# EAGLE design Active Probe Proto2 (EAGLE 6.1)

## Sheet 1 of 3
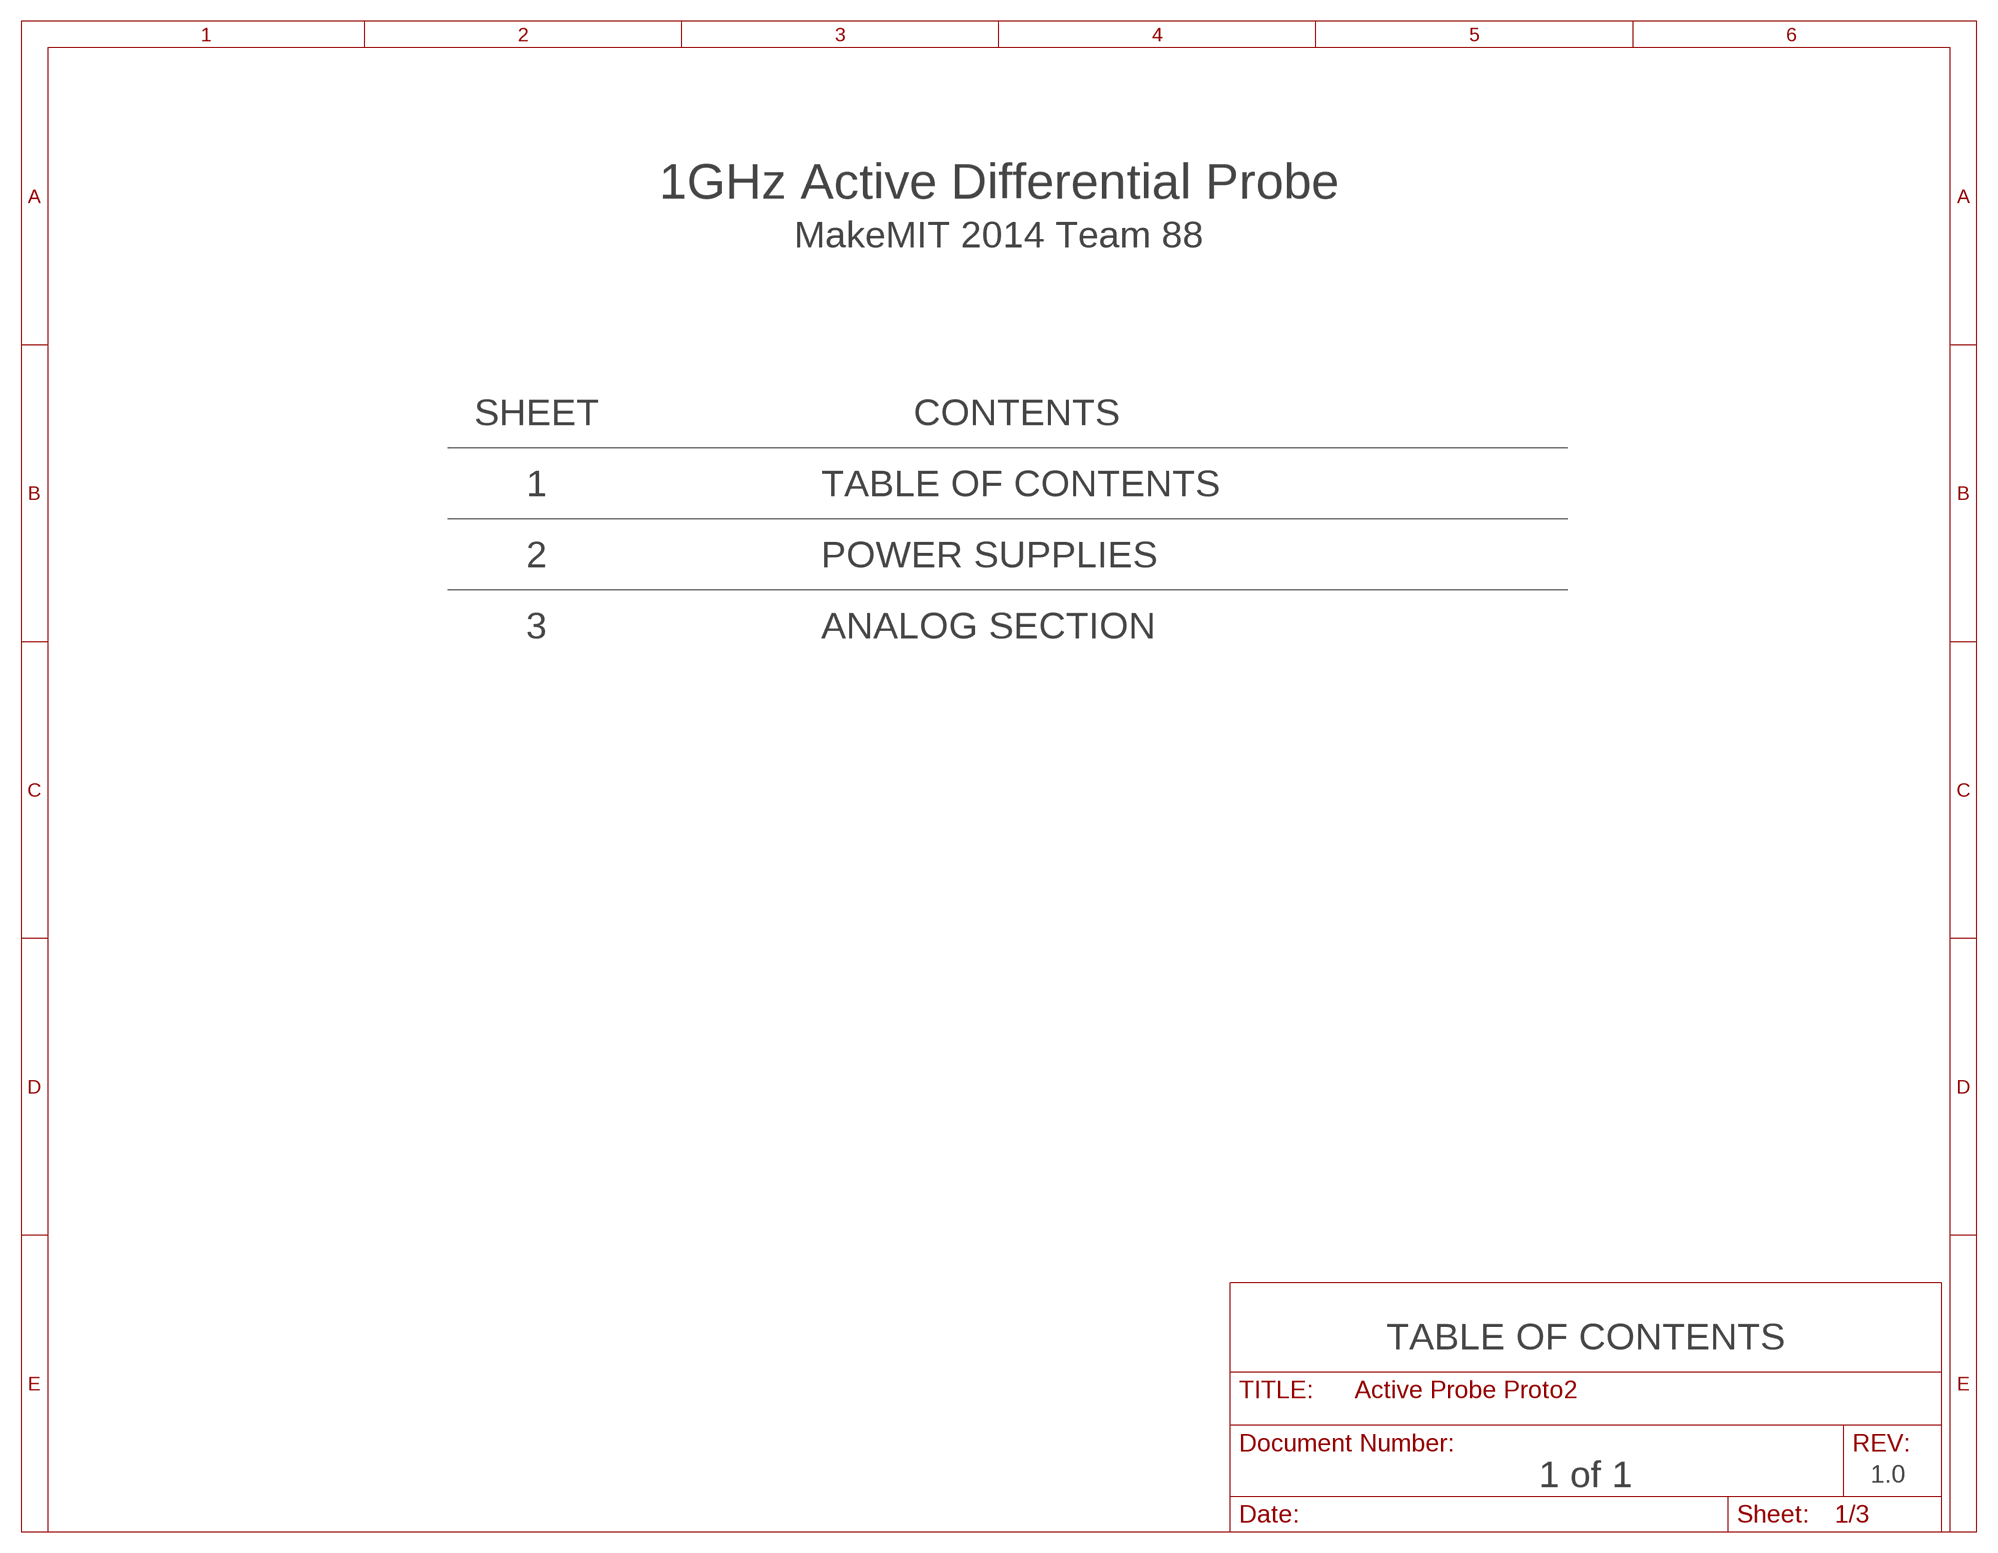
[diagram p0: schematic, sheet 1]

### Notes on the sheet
- 1GHz Active Differential Probe
- MakeMIT 2014 Team 88
- SHEET | CONTENTS
- 1 | TABLE OF CONTENTS
- 2 | POWER SUPPLIES
- 3 | ANALOG SECTION
- TABLE OF CONTENTS
- 1 of 1 | 1.0

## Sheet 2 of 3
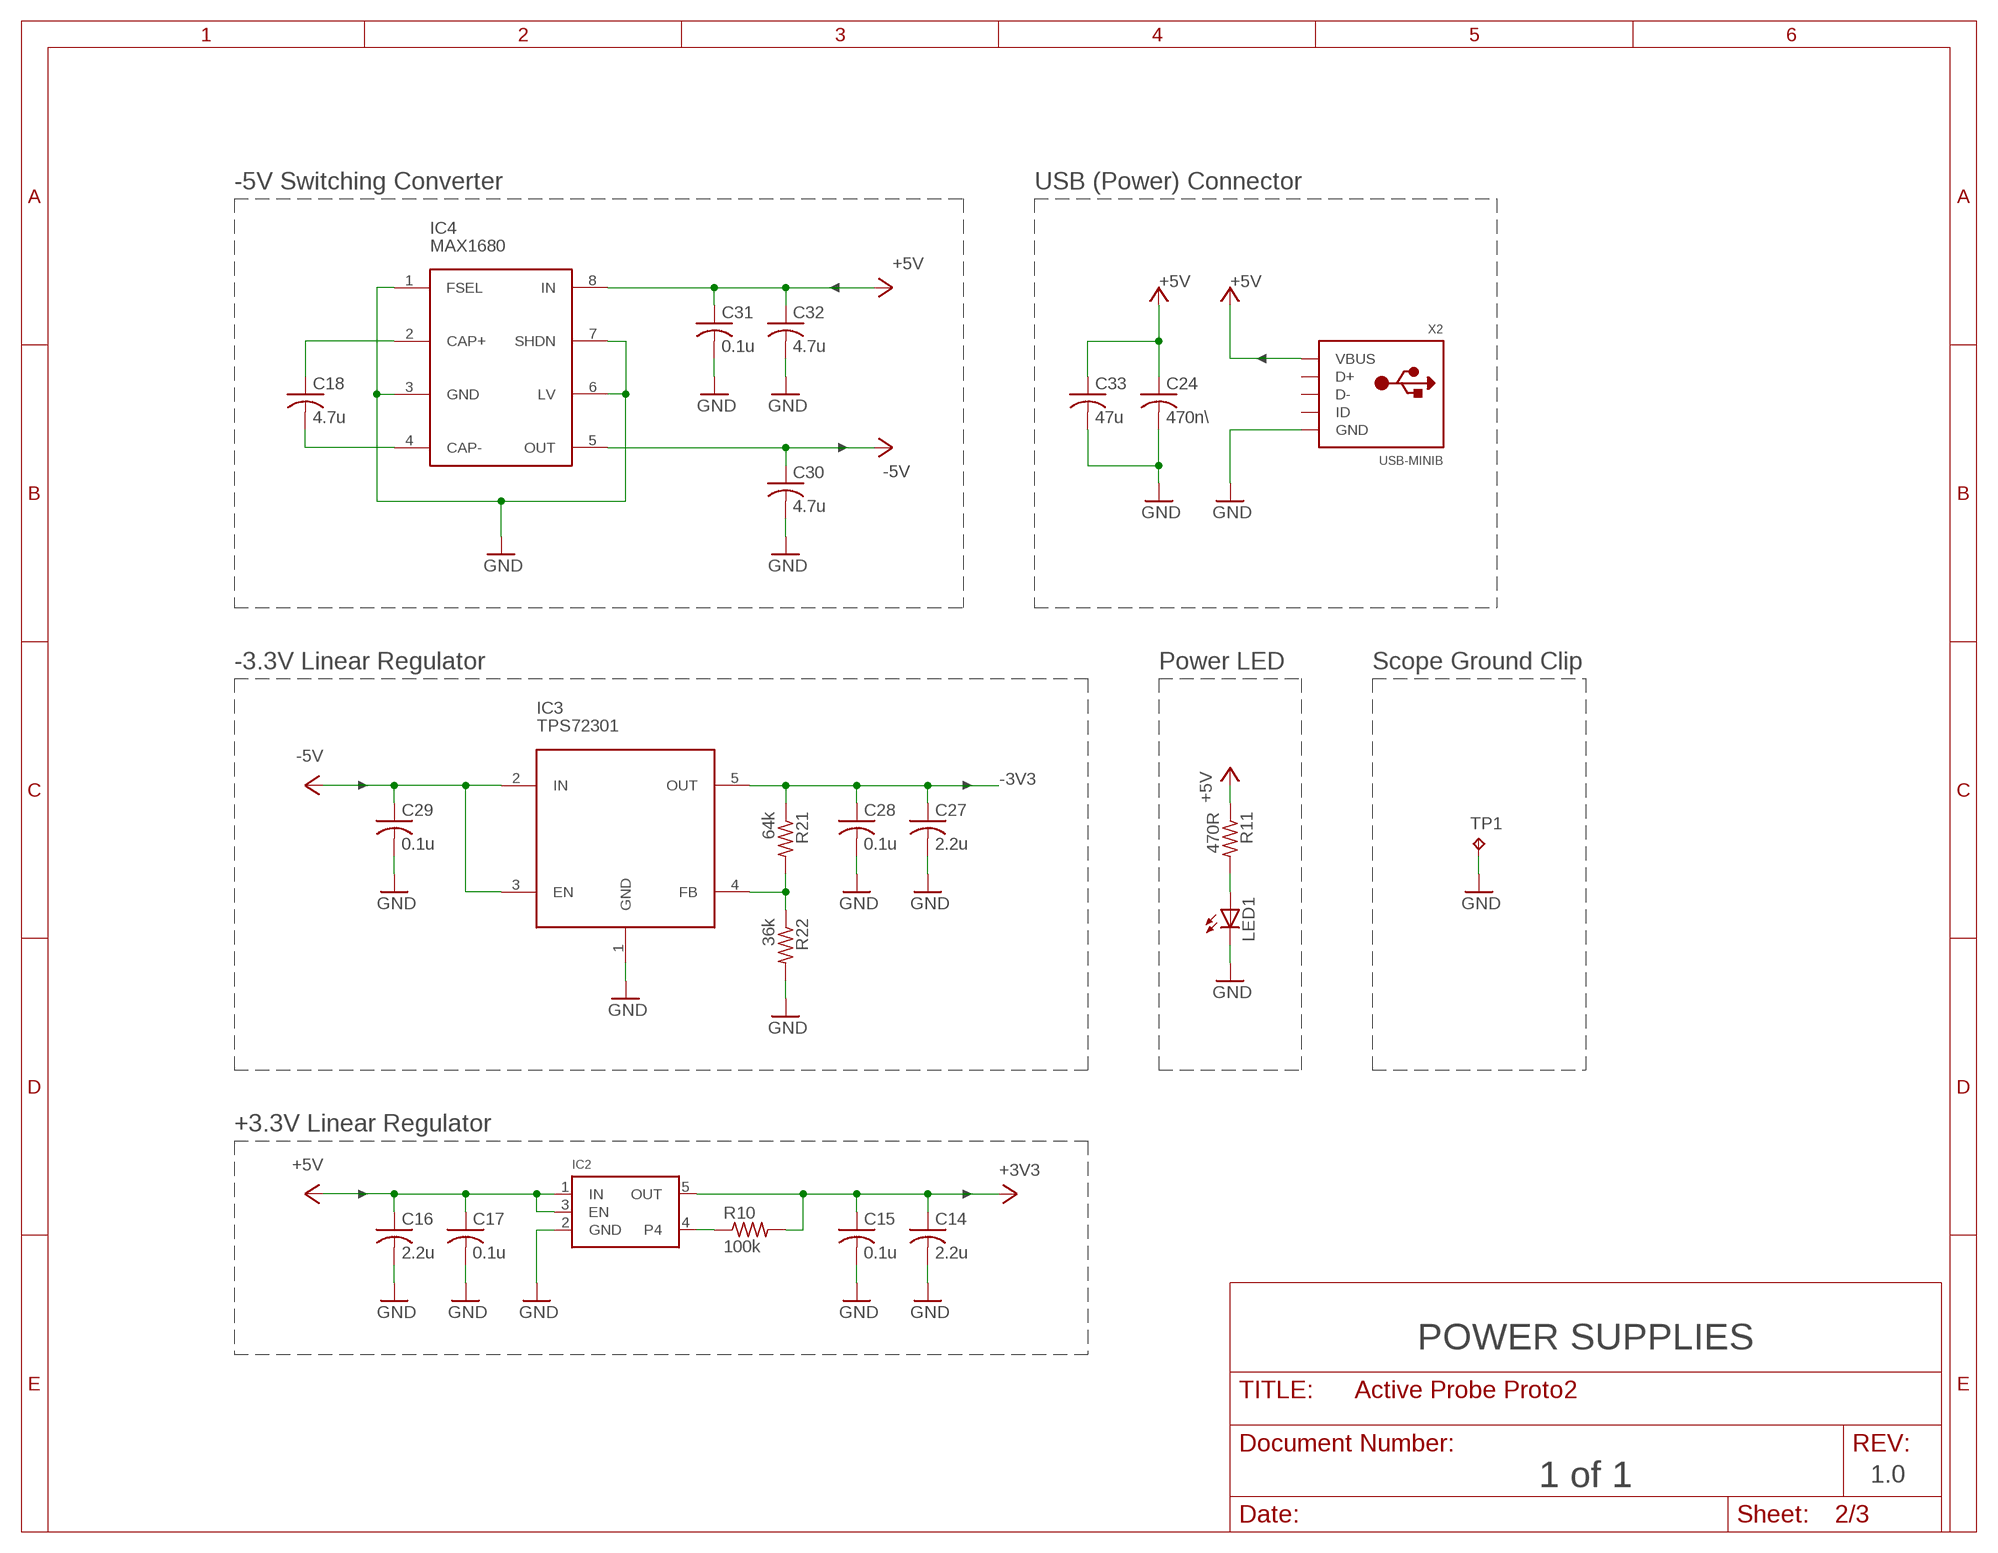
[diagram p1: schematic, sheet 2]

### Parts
C14  2.2u  C-USC0603  [C0603]
C15  0.1u  C-USC0603  [C0603]
C16  2.2u  C-USC0603  [C0603]
C17  0.1u  C-USC0603  [C0603]
C18  4.7u  C-USC0603  [C0603]
C24  470n\  C-USC0603  [C0603]
C27  2.2u  C-USC0603  [C0603]
C28  0.1u  C-USC0603  [C0603]
C29  0.1u  C-USC0603  [C0603]
C30  4.7u  C-USC0603  [C0603]
C31  0.1u  C-USC0603  [C0603]
C32  4.7u  C-USC0603  [C0603]
C33  47u  C-USC1206  [C1206]
IC2  VREG_SOT23-5  [SOT23-5]
IC3  TPS72301  [SOT23-5L]
IC4  MAX1680  MAX1680/1  [SO8]
LED1  LED3MM  [LED3MM]
R10  100k  R-US_R0603  [R0603]
R11  470R  R-US_R0805  [R0805]
R21  64k  R-US_R0603  [R0603]
R22  36k  R-US_R0603  [R0603]
TP1  TPTP20SQ  [TP20SQ]
X2  USB-MINIB  USBMINIB  [USB-MINIB]

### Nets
+3V3: C14.1 C15.1 IC2.5(OUT) R10.2 ; also sheet 3
+5V: C16.1 C17.1 C24.1 C31.1 C32.1 C33.1 IC2.1(IN) IC2.3(EN) IC4.8(IN) R11.1 X2.VBUS ; also sheet 3
-3V3: C27.1 C28.1 IC3.5(OUT) R21.1 ; also sheet 3
-5V: C29.1 C30.1 IC3.2(IN) IC3.3(EN) IC4.5(OUT)
GND: C14.2 C15.2 C16.2 C17.2 C24.2 C27.2 C28.2 C29.2 C30.2 C31.2 C32.2 C33.2 IC2.2(GND) IC3.1(GND) IC4.1(FSEL) IC4.3(GND) IC4.6(LV) IC4.7(SHDN) LED1.K(C) R22.2 TP1.TP X2.GND ; also sheet 3
N$4: IC2.4 R10.1
N$11: LED1.A R11.2
N$14: C18.2 IC4.4(CAP-)
N$15: C18.1 IC4.2(CAP+)
N$19: IC3.4(FB) R21.2 R22.1
Unconnected: X2.D+ X2.D- X2.ID

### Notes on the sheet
- -5V Switching Converter | USB (Power) Connector
- -3.3V Linear Regulator | Power LED | Scope Ground Clip
- +3.3V Linear Regulator
- POWER SUPPLIES
- 1 of 1 | 1.0

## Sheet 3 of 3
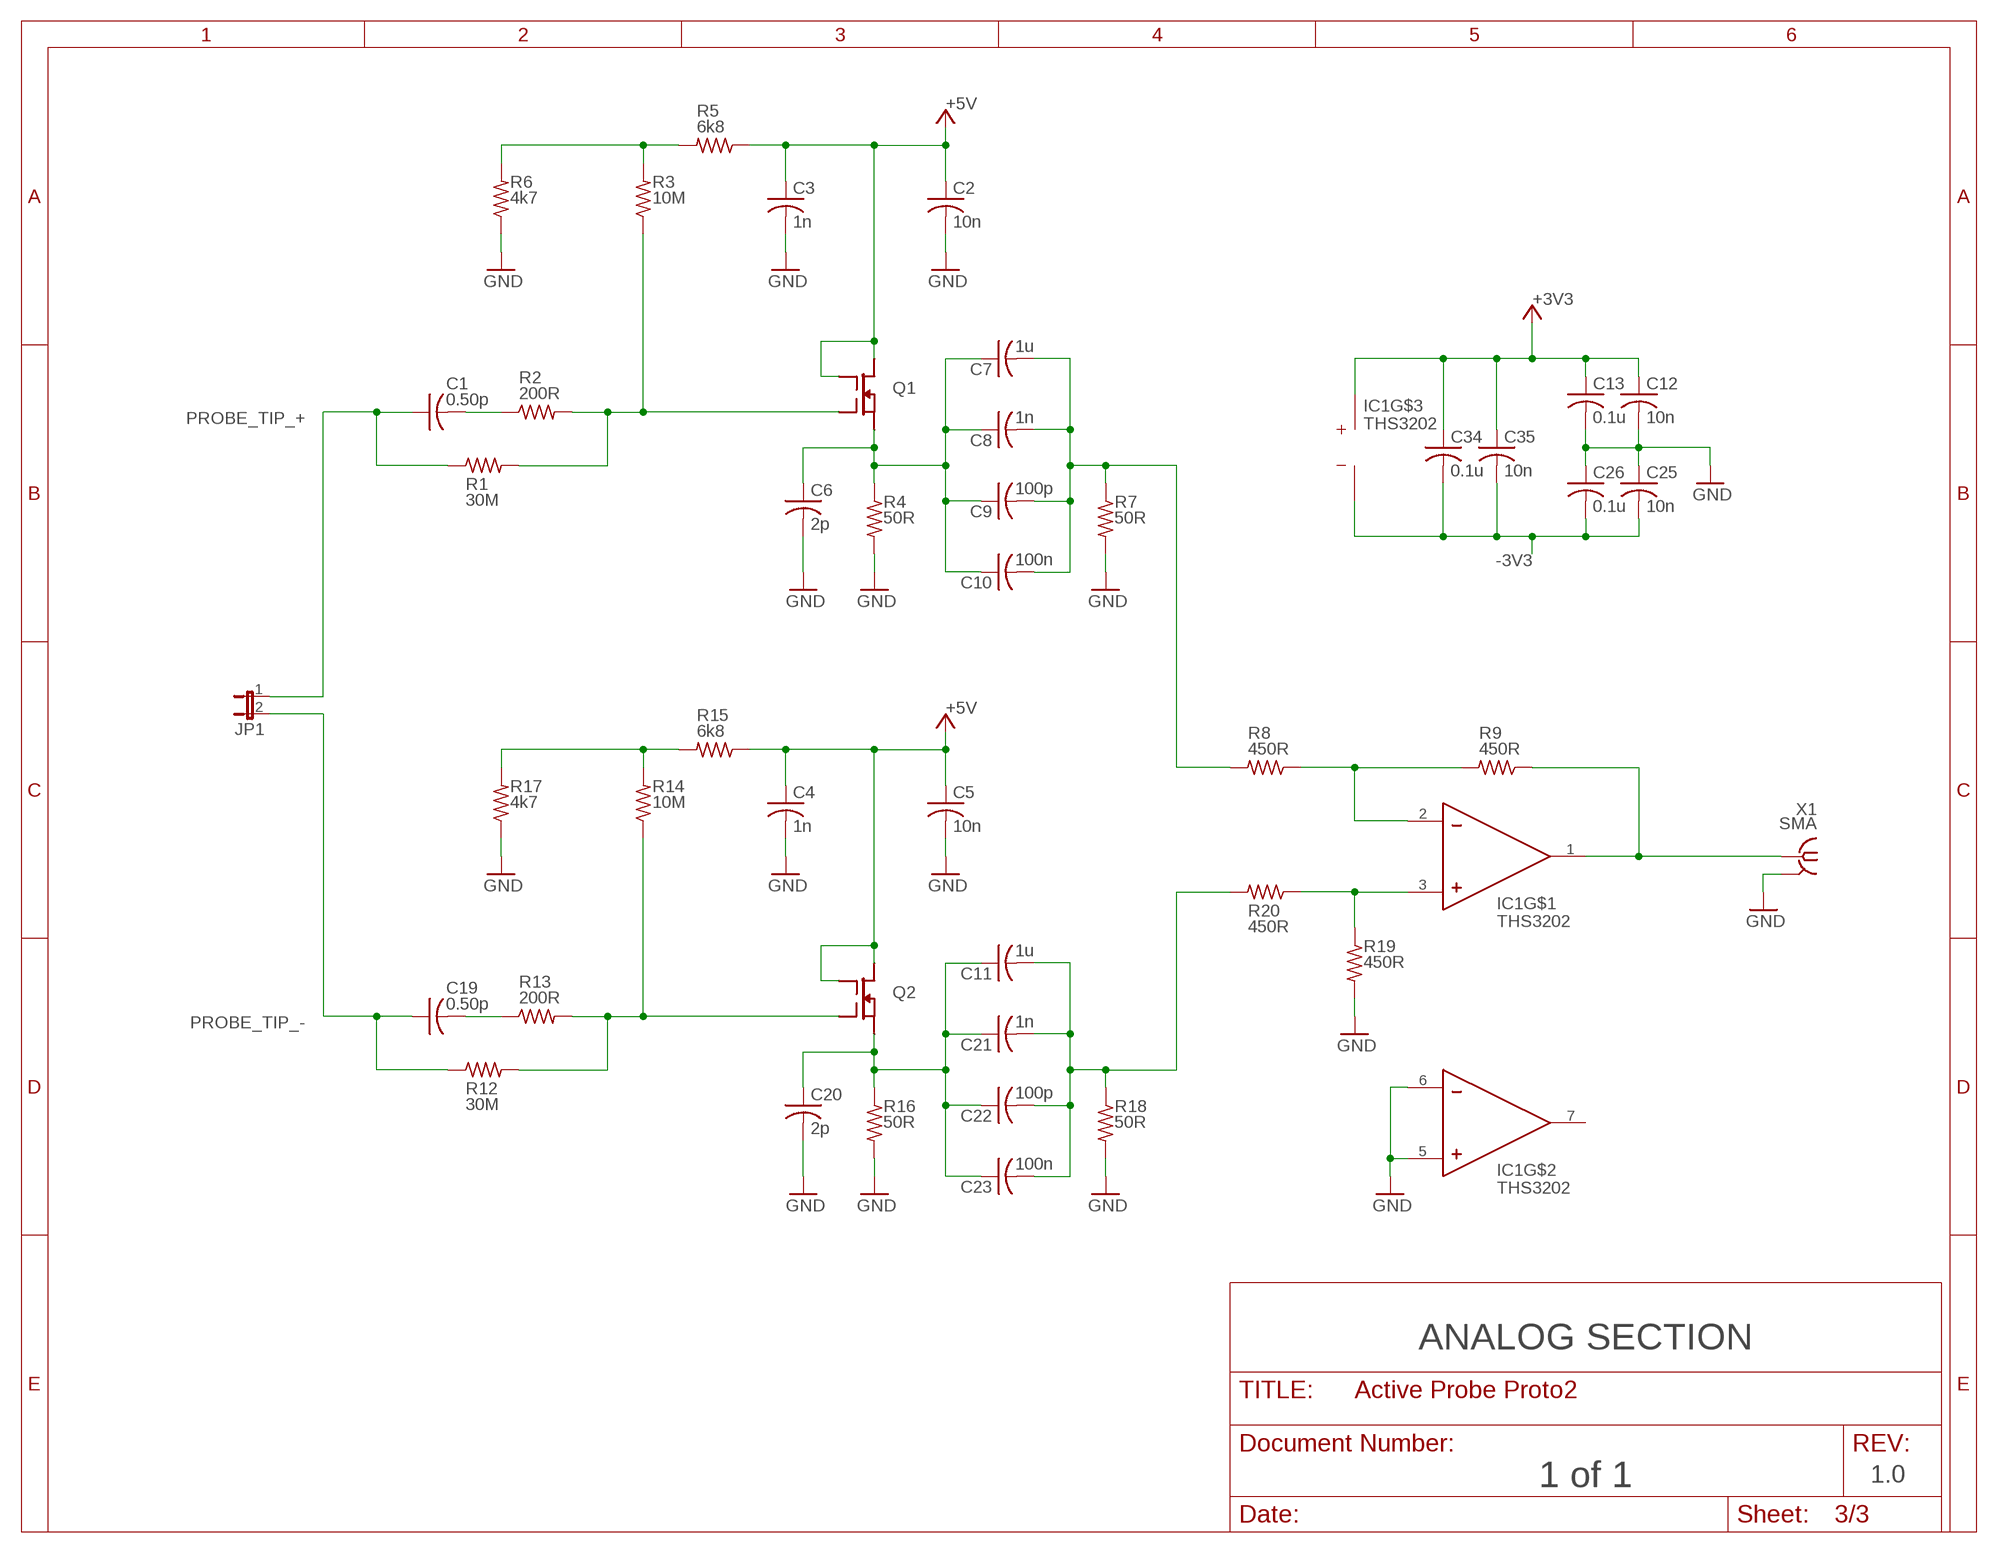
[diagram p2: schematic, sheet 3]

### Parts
C1  0.50p  C-USC0603  [C0603]
C2  10n  C-USC0603  [C0603]
C3  1n  C-USC0603  [C0603]
C4  1n  C-USC0603  [C0603]
C5  10n  C-USC0603  [C0603]
C6  2p  C-USC0603  [C0603]
C7  1u  C-USC0603  [C0603]
C8  1n  C-USC0603  [C0603]
C9  100p  C-USC0603  [C0603]
C10  100n  C-USC0603  [C0603]
C11  1u  C-USC0603  [C0603]
C12  10n  C-USC0603  [C0603]
C13  0.1u  C-USC0603  [C0603]
C19  0.50p  C-USC0603  [C0603]
C20  2p  C-USC0603  [C0603]
C21  1n  C-USC0603  [C0603]
C22  100p  C-USC0603  [C0603]
C23  100n  C-USC0603  [C0603]
C25  10n  C-USC0603  [C0603]
C26  0.1u  C-USC0603  [C0603]
C34  0.1u  C-USC0603  [C0603]
C35  10n  C-USC0603  [C0603]
IC1  THS3202  [SOIC8]
JP1  HEADER_SIDE_2POS  [HEADER_SIDE_2POS]
Q1  BF998  [SOT143B]
Q2  BF998  [SOT143B]
R1  30M  R-US_R0603  [R0603]
R2  200R  R-US_R0603  [R0603]
R3  10M  R-US_R0603  [R0603]
R4  50R  R-US_R0603  [R0603]
R5  6k8  R-US_R0603  [R0603]
R6  4k7  R-US_R0603  [R0603]
R7  50R  R-US_R0603  [R0603]
R8  450R  R-US_R0603  [R0603]
R9  450R  R-US_R0603  [R0603]
R12  30M  R-US_R0603  [R0603]
R13  200R  R-US_R0603  [R0603]
R14  10M  R-US_R0603  [R0603]
R15  6k8  R-US_R0603  [R0603]
R16  50R  R-US_R0603  [R0603]
R17  4k7  R-US_R0603  [R0603]
R18  50R  R-US_R0603  [R0603]
R19  450R  R-US_R0603  [R0603]
R20  450R  R-US_R0603  [R0603]
X1  SMA  SMA-142-0701-801/806  [J502-ND-142-0701-801/806]

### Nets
+3V3: C12.1 C13.1 C34.1 C35.1 IC1.8(VCC) ; also sheet 2
+5V: C2.1 C3.1 C4.1 C5.1 Q1.2(D) Q1.3(G2) Q2.2(D) Q2.3(G2) R5.1 R15.1 ; also sheet 2
-3V3: C25.2 C26.2 C34.2 C35.2 IC1.4(GND) ; also sheet 2
GND: C2.2 C3.2 C4.2 C5.2 C6.2 C12.2 C13.2 C20.2 C25.1 C26.1 IC1.5(IN+) IC1.6(IN-) R4.2 R6.1 R7.2 R16.2 R17.1 R18.2 R19.2 X1.G@1(GND) ; also sheet 2
N$1: R14.2 R15.2 R17.2
N$2: C6.1 C7.1 C8.1 C9.1 C10.1 Q1.1(S) R4.1
N$3: R3.2 R5.2 R6.2
N$5: C7.2 C8.2 C9.2 C10.2 R7.1 R8.2
N$6: Q1.4(G1) R1.2 R2.2 R3.1
N$7: C11.2 C21.2 C22.2 C23.2 R18.1 R20.2
N$8: Q2.4(G1) R12.2 R13.2 R14.1
N$9: C11.1 C20.1 C21.1 C22.1 C23.1 Q2.1(S) R16.1
N$12: C19.2 R13.1
N$13: IC1.1(OUT) R9.1 X1.1
N$16: IC1.3(IN+) R19.1 R20.1
N$17: IC1.2(IN-) R8.1 R9.2
N$18: C1.2 R2.1
PROBE_TIP_+: C1.1 JP1.1 R1.1
PROBE_TIP_-: C19.1 JP1.2 R12.1
Unconnected: IC1.7(OUT)

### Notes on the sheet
- ANALOG SECTION
- 1 of 1 | 1.0

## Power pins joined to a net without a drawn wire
GND: X1.G@2(GND) X1.G@3(GND) X1.G@4(GND)

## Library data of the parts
C1-C35 = rcl:C-US: CAPACITOR, American symbol
IC1 = Kramnik's Library:THS3202
IC2 = microbuilder:VREG_SOT23-5: SOT23-5 Fixed Voltage Regulators To better organise some of the SOT23-5 fixed voltage regulators in this library, this new part was created. Part Current Out V Out V In V Dropout Digikey Part No. ADP121 150mA 3.3V 3.4-5.5V 0.09V @ 150mA ADP121-AUJZ33R7CT-ND ADP121 150mA 3.0V 3.1-5.5V 0.09V @ 150mA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
IC3 = Kramnik's Library:TPS72301
IC4 = Kramnik's Library:MAX1680/1: 125mA, Frequency-Selectable, Switched-Capacitor Voltage Converter Digikey: http://www.digikey.com/product-detail/en/MAX1681ESA%2B/MAX1681ESA%2B-ND/947772
JP1 = Kramnik's Library:HEADER_SIDE_2POS
LED1 = led:LED: LED
Q1 Q2 = Kramnik's Library:BF998
R1-R22 = resistor:R-US_: RESISTOR, American symbol
TP1 = testpad:TP: Test pad
X1 = con-coax:SMA-: SMA 50 Ohm End Launch Jack Receptacle - Round Contact Johnson Components Source: www.johnsoncomponents.com .. J502-ND.pdf; MF: JOHNSON COMPONENTS; MPN: 142-0701-801; OC_FARNELL: 1608592; OC_NEWARK: 90F2624
X2 = adafruit:USB: USB Connectors USBMINIB - Surface Mount Female Mini-B USB Connector 4UConnector: 06564 By microbuilder.eu Thru-hole RA Female Mini-B USB Connector 4UConnector: 18732 By ladyada.net

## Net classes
1 Power: width 0.305 mm, drill 0.381 mm, clearance 0.203 mm
2 50OHM_SE: width 0.229 mm, drill 0.381 mm, clearance 0.203 mm

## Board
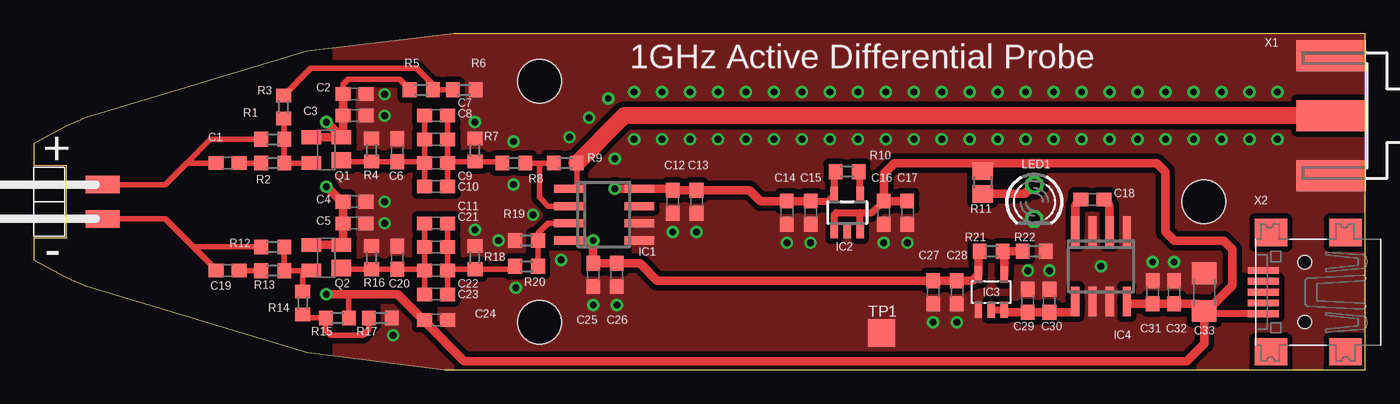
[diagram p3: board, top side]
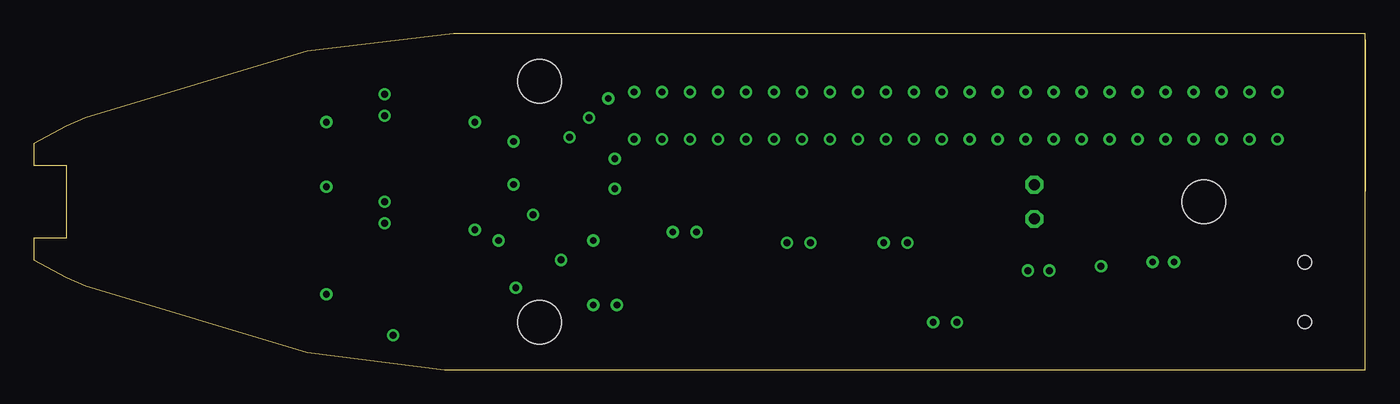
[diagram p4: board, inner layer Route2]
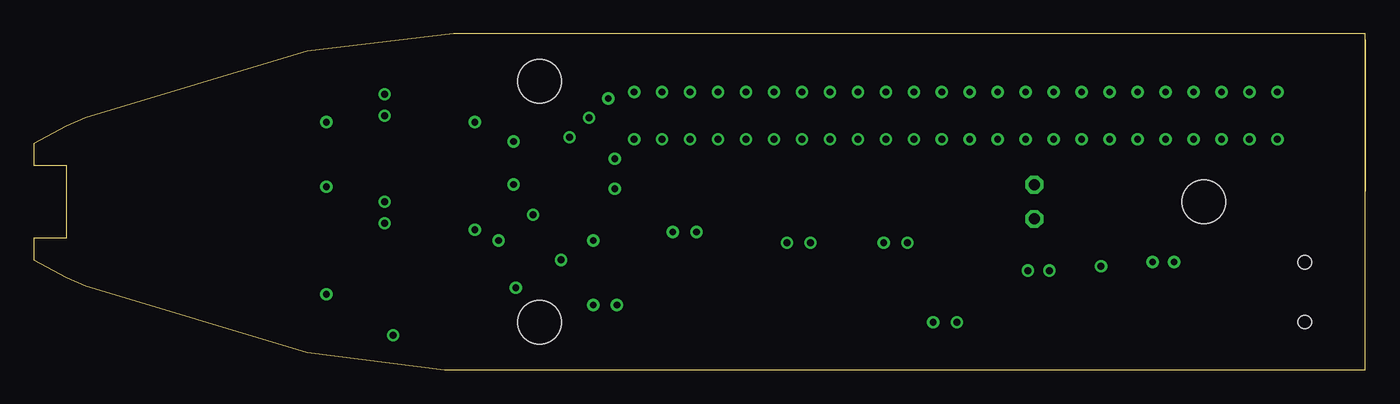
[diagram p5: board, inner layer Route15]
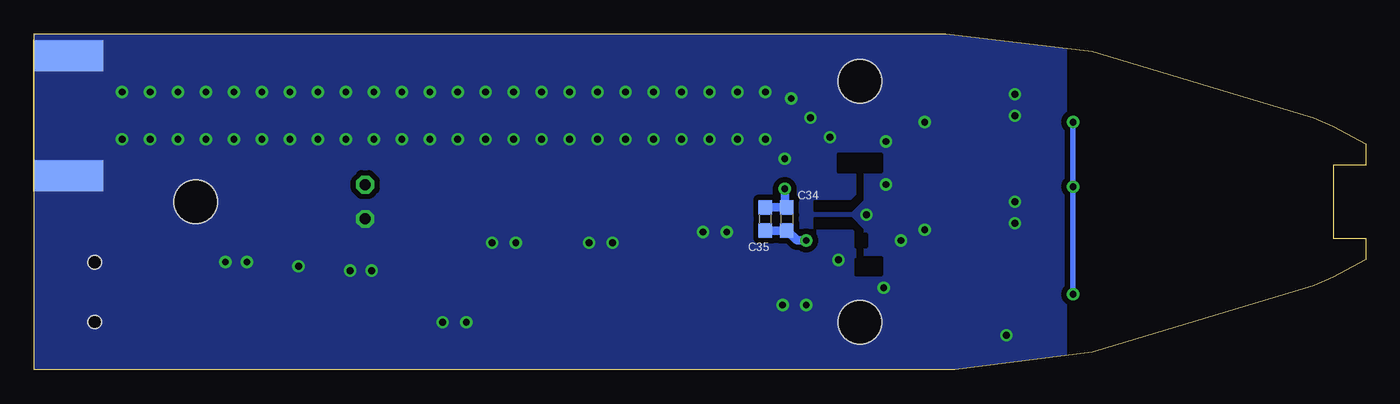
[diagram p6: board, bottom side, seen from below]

Size 98.27 x 24.77 mm. Coordinates in mm from the lower left corner, seen from the top.
Outline: 20.16,1.27 30.32,0 98.25,0 98.25,24.77 30.96,24.77 20.16,23.5 3.81,18.57 2.38,17.94 0,16.67 0,15.08 2.38,15.08 2.38,9.68 0,9.68 0,8.1 2.38,6.83 3.81,6.19 20.16,1.27
Copper layers (1*16): Top 0.035mm / dielectric 1.5mm / Bottom 0.035mm
Design rules: minimum track width 10mil, minimum drill 24mil, track to track 16mil, track to pad 16mil, pad to pad 16mil, via to via 16mil, smd to smd 1mil, copper to edge 1mil, drill to drill 8mil, minimum pad ring 10mil, minimum via ring 8mil, stop-mask expansion 4mil, vias tented up to drill 0mil, thermal gap 10mil
Holes 3.2 mm at 86.33,12.38 37.31,21.27 37.31,3.49
tRestrict: area 40.2,8.9 to 44,14
bRestrict: area 35.7,11.7 to 40.6,15.9; area 35.7,7 to 40.6,11.1

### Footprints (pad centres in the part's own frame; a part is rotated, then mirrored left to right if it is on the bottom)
C0603 = smd 1.1 x 1: 1 -0.85,0; 2 0.85,0
C1206 = smd 1.6 x 1.8: 1 -1.4,0; 2 1.4,0
SOIC8 = smd 0.6 x 2.2: 1 -1.905,-2.6; 2 -0.635,-2.6; 3 0.635,-2.6; 4 1.905,-2.6; 5 1.905,2.6; 6 0.635,2.6; 7 -0.635,2.6; 8 -1.905,2.6
SOT23-5 = smd 0.55 x 1.2: 1 -0.95,-1.3; 2 0,-1.3; 3 0.95,-1.3; 4 0.95,1.3; 5 -0.95,1.3
SOT23-5L = smd 0.55 x 1.2: 1 -0.95,-1.3; 2 0,-1.3; 3 0.95,-1.3; 4 0.95,1.3; 5 -0.95,1.3
SO8 = smd 0.6 x 2.2: 1 -1.905,-2.6; 2 -0.635,-2.6; 3 0.635,-2.6; 4 1.905,-2.6; 5 1.905,2.6; 6 0.635,2.6; 7 -0.635,2.6; 8 -1.905,2.6
HEADER_SIDE_2POS = smd 2.54 x 1.27: 1 5.08,3.81; 2 5.08,1.27
LED3MM = drill 0.813 octagon: A -1.27,0; K 1.27,0
SOT143B = smd 1.2 x 1.44: 1 -0.75,-1.1 | smd 1 x 1.44: 2 0.95,-1.1; 3 0.95,1.1; 4 -0.95,1.1
R0603 = smd 1 x 1.1: 1 -0.85,0; 2 0.85,0
R0805 = smd 1.3 x 1.5: 1 -0.85,0; 2 0.85,0
TP20SQ = smd 2 x 2: TP 0,0
J502-ND-142-0701-801/806 = smd 5.08 x 2.286: 1 2.565,0; G@1 2.565,4.42; G@2 2.565,-4.42 | smd 5.08 x 2.286 bottom: G@3 2.565,4.42; G@4 2.565,-4.42
USB-MINIB = smd 0.5 x 2.308: D+ 0,4.064; D- -0.8,4.064; GND 1.6,4.064; ID 0.8,4.064; VBUS -1.6,4.064 | smd 2 x 2.4: GND1 -4.4,-2; GND2 -4.4,3.5; GND3 4.4,3.5; GND4 4.4,-2 | hole 1: -2.2,1; 2.2,1

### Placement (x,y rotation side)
C1  14.29,15.24 0 top
C2  23.65,20.32 0 top
C3  23.65,18.73 0 top
C4  23.65,12.38 0 top
C5  23.65,10.79 0 top
C6  26.83,16.19 90 top
C7  29.69,18.73 0 top
C8  29.69,16.99 0 top
C9  29.69,15.24 0 top
C10  29.69,13.49 0 top
C11  29.69,10.79 0 top
C12  47.15,12.38 270 top
C13  48.89,12.38 270 top
C14  55.56,11.59 270 top
C15  57.31,11.59 270 top
C16  62.71,11.59 270 top
C17  64.45,11.59 270 top
C18  78.11,12.54 180 top
C19  14.29,7.3 0 top
C20  26.83,8.26 90 top
C21  29.69,9.05 0 top
C22  29.69,7.3 0 top
C23  29.69,5.56 0 top
C24  29.69,3.65 0 top
C25  41.27,6.99 90 top
C26  43.02,6.99 90 top
C27  66.36,5.71 270 top
C28  68.1,5.71 270 top
C29  73.34,5.08 90 top
C30  74.93,5.08 90 top
C31  82.55,5.71 90 top
C32  84.14,5.71 90 top
C33  86.36,5.71 90 top
C34  42.7,11.11 270 bottom
C35  44.29,11.11 270 bottom
IC1  42.07,11.43 270 top
IC2  60.01,11.59 0 top
IC3  70.64,5.71 0 top
IC4  78.74,7.62 180 top
JP1  0,9.84 0 top
LED1  73.82,12.38 270 top
Q1  21.59,16.19 90 top
Q2  21.59,8.26 90 top
R1  17.62,16.99 0 top
R2  17.62,15.24 0 top
R3  18.42,19.37 90 top
R4  24.92,16.19 90 top
R5  28.58,20.64 0 top
R6  31.75,20.64 180 top
R7  32.54,16.19 90 top
R8  35.4,15.24 180 top
R9  39.21,15.24 180 top
R10  60.01,14.61 180 top
R11  70.01,13.81 270 top
R12  17.62,9.05 0 top
R13  17.62,7.3 0 top
R14  19.84,4.92 270 top
R15  22.38,3.81 180 top
R16  24.92,8.26 90 top
R17  25.56,3.81 180 top
R18  32.54,8.26 90 top
R19  36.35,9.53 180 top
R20  36.35,7.62 180 top
R21  70.64,8.73 0 top
R22  73.82,8.73 0 top
TP1  62.55,2.7 0 top
X1  98.27,18.73 180 top
X2  94.77,5.71 90 top

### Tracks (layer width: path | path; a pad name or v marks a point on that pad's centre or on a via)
+3V3  (via drill 0.5)
  Top 0.508: C15.1 58.61,12.44 IC2.5 59.06,14.51 R10.2
  Top 0.61: v42.86,13.34 IC1.8 47.05,13.34 C12.1 C13.1 52.81,13.23 53.6,12.44 C14.1 C15.1
  Bottom 0.61: C35.1 C34.1 42.86,12.12 v42.86,13.34
+5V  (via drill 0.5)
  Top 0.254: 22.86,9.21 Q2.2
  Top 0.406: R15.1 23.23,5.5 23.18,5.56 | C24.1 28.84,3.6 28.81,3.57 | R5.1 27.73,20.69 26.99,21.43 23.18,21.43 22.8,21.06 C2.1
  Top 0.508: X2.VBUS 86.56,4.12 C33.1 | IC2.1 59.06,11.43 59.21,11.59 60.96,11.59 | IC2.3 60.96,11.59 | 60.96,11.59 61.85,11.59 C16.1
  Top 0.61: Q2.3 Q2.2 22.8,9.32 C5.1 C4.1 22.7,12.38 v21.59,13.49 | Q1.3 Q1.2 | Q1.2 22.8,17.26 C3.1 C2.1 | IC4.8 80.8,4.87 C31.1 C32.1 85.81,4.87 C33.1 86.36,4.13 | C17.1 C16.1 62.71,14.45 63.5,15.24 70.01,15.24 | v21.59,18.26 21.59,18.24 Q1.2 | 86.36,4.13 86.36,1.91 85.09,0.64 31.75,0.64 28.81,3.57 26.83,5.56 23.18,5.56 v21.59,5.56 | 70.01,15.24 82.87,15.24 83.5,14.61 83.5,10.16 84.14,9.53 87.79,9.53 88.42,8.89 88.42,6.19 86.36,4.13 | R11.1 70.01,15.24
  Bottom 0.406: v21.59,18.26 v21.59,13.49 v21.59,5.56
-3V3  (via drill 0.5)
  Top 0.61: IC1.4 v41.28,9.53 C25.2 C26.2 44.71,7.83 45.98,6.57 C27.1 C28.1 69.24,6.57 IC3.5 69.69,8.63 R21.1
  Bottom 0.508: v41.28,9.53
  Bottom 0.61: C35.2 C34.2 41.97,9.53 v41.28,9.53
-5V
  Top 0.508: IC3.2 IC3.3
  Top 0.61: IC3.3 71.78,4.23 C29.1 C30.1 76.62,4.23 76.84,4.45 IC4.5
GND  (via drill 0.5)
  other vias: 91.76,20.48 91.76,16.99 78.74,7.62 25.88,18.73 82.55,7.94 47.15,10.16 48.89,10.16 43.02,4.76 41.27,4.76 74.93,7.3 89.69,16.99 89.69,20.48 87.63,20.48 87.63,16.99 85.57,16.99 85.57,20.48 83.5,20.48 83.5,16.99 81.44,16.99 81.44,20.48 79.38,20.48 79.38,16.99 77.31,16.99 77.31,20.48 75.25,16.99 75.25,20.48 73.18,20.48 73.18,16.99 71.12,16.99 71.12,20.48 69.06,20.48 69.06,16.99 66.99,16.99 66.99,20.48 64.93,20.48 64.93,16.99 62.87,16.99 62.87,20.48 60.8,20.48 60.8,16.99 58.74,16.99 58.74,20.48 56.67,20.48 56.67,16.99 54.61,16.99 54.61,20.48 52.55,20.48 52.55,16.99 50.48,16.99 50.48,20.48 48.42,16.99 48.42,20.48 46.35,20.48 46.35,16.99 44.29,16.99 44.29,20.48 42.39,20 40.96,18.57 39.53,17.14 42.86,15.56 25.88,20.32 25.88,10.79 25.88,12.38 84.14,7.94 73.34,7.3 68.1,3.49 66.36,3.49 55.56,9.37 57.31,9.37 62.71,9.37 64.45,9.37 38.89,8.1 36.83,11.43 34.29,9.53 32.54,10.32 32.54,18.26 26.51,2.54 35.4,16.83 35.4,13.65 35.56,6.03
  pour Top (no thermals): 98.9,28.57 22.22,28.89 22.22,-3.81 98.9,-3.49
  pour Bottom (no thermals): 98.9,28.26 98.9,-3.17 22.22,-3.81 22.22,28.26
  pour Route2: -5.87,-10.16 72.87,-10.16 72.87,-86.36 -5.87,-86.36
  pour Route15: 36.35,-10.48 56.36,-10.48 56.99,-11.11 56.99,-24.45 55.72,-25.72 55.72,-28.26 62.39,-34.92 62.39,-40.01 61.75,-40.64 36.04,-40.64 34.45,-39.05 34.45,-20.64 35.72,-19.37 35.72,-11.11
N$1
  Top 0.406: R17.2 24.71,2.96 24.29,2.54 21.91,2.54 21.53,2.91 R15.2 20.11,3.81 R14.2
N$2
  Top 0.406: Q1.1 22.79,15.34 R4.1 C6.1 28.73,15.34 C9.1 | C9.1 C8.1 C7.1 | C10.1 C9.1
N$3
  Top 0.406: R6.2 R5.2 29.43,21.06 28.26,22.23 20.42,22.23 R3.2
N$4
  Top 0.508: IC2.4 60.96,14.51 R10.1
N$5
  Top 0.406: C9.2 C8.2 C7.2 | C9.2 30.64,15.34 R7.1 34.45,15.34 R8.2 | C10.2 C9.2
N$6
  Top 0.406: Q1.4 R2.2 R1.2 18.47,18.46 R3.1
N$7
  Top 0.406: C22.2 C21.2 C11.2 | C22.2 30.64,7.41 R18.1 35.29,7.41 R20.2 | C23.2 C22.2
N$8
  Top 0.406: R12.2 R13.2 19.84,7.3 | 19.84,7.3 Q2.4 | R14.1 19.84,7.3
N$9
  Top 0.406: Q2.1 22.79,7.41 R16.1 C20.1 28.73,7.41 C22.1 | C22.1 C21.1 C11.1 | C23.1 C22.1
N$11
  Top 0.61: R11.2 73.13,12.96 LED1.A
N$12
  Top 0.406: R13.1 C19.2
N$13
  Top 0.406: R9.1 40.06,13.34 IC1.1
  Top 1.27: X1.1 43.55,18.73 R9.1
N$14
  Top 0.61: IC4.4 76.84,12.12 C18.2
N$15
  Top 0.61: IC4.2 79.38,12.12 C18.1
N$16
  Top 0.406: IC1.3 37.94,10.79 37.2,10.06 R19.1 R20.1
N$17
  Top 0.406: R9.2 37.31,15.24 | 37.31,15.24 R8.1 | IC1.2 37.94,12.06 37.31,12.7 37.31,15.24
N$18
  Top 0.406: R2.1 C1.2
N$19
  Top 0.61: R22.1 R21.2 71.59,8.63 IC3.4
PROBE_TIP_+
  Top 0.406: R1.1 13.02,16.99 11.27,15.24 | 11.27,15.24 C1.1 | JP1.1 9.68,13.65 11.27,15.24
PROBE_TIP_-
  Top 0.406: JP1.2 9.68,11.11 11.67,9.13 11.75,9.05 | C19.1 13.44,7.36 11.75,9.05 | R12.1 11.75,9.05

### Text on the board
tNames: 1GHz Active Differential Probe | + | -

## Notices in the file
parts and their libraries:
microbuilder: This work is placed in the public domain, and may be freely used for commercial and non-commercial work with the following conditions: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
